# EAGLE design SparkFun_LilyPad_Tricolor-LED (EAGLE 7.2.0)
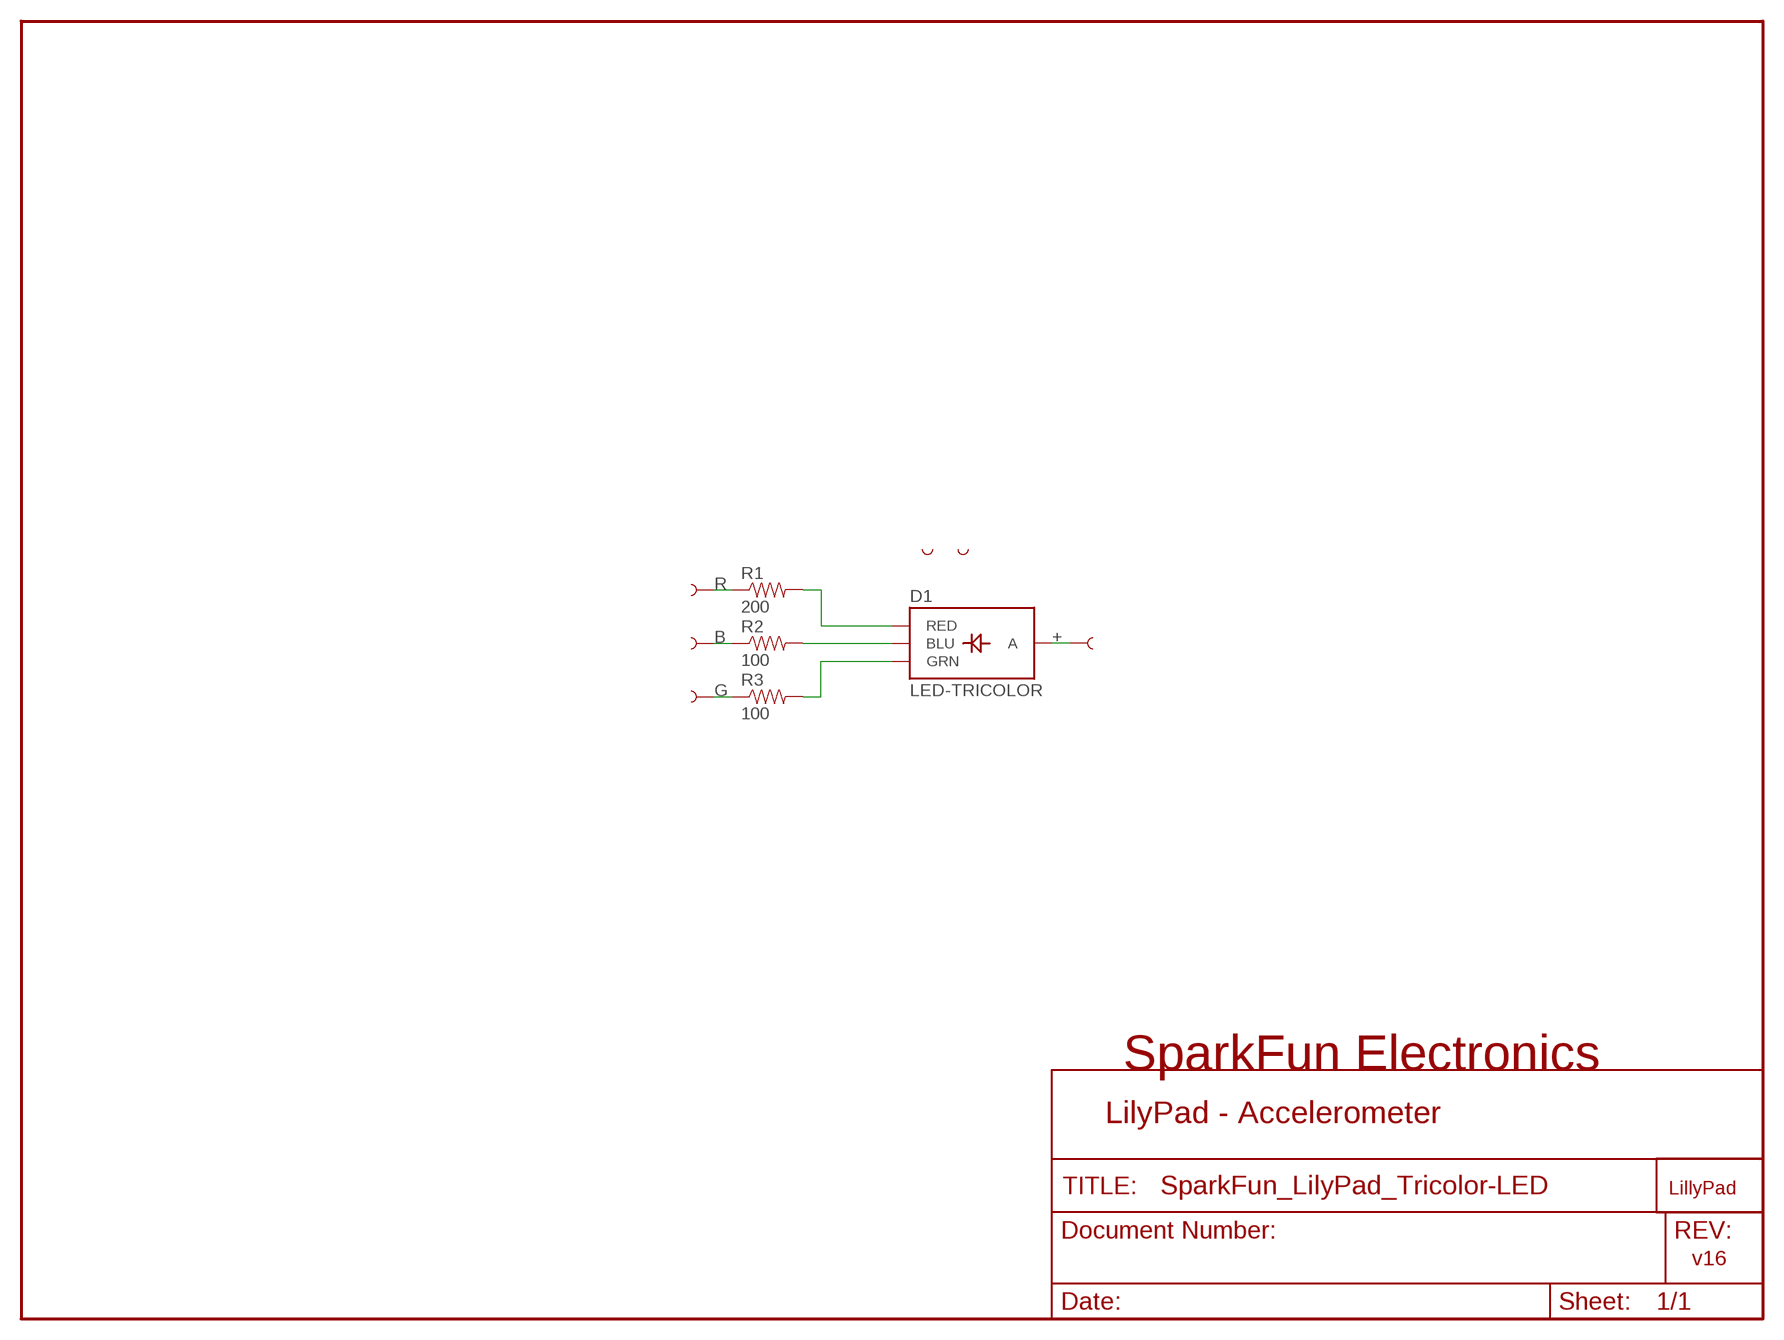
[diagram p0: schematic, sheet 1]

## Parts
D1  LED-TRICOLOR  [LED-TRICOLOR-SMD]
R1  200  RESISTOR0402-RES  [0402-RES]
R2  100  RESISTOR0402-RES  [0402-RES]
R3  100  RESISTOR0402-RES  [0402-RES]
U$1  LOGO-LPL  [LOGO-L]
U$2  SEWTAP-NOHOLE2  [PETAL-NOHOLE-2SIDE]
U$3  SEWTAP-NOHOLE2  [PETAL-NOHOLE-2SIDE]
U$7  SEWTAP6  [PETAL-SMALL-2SIDE]
U$8  SEWTAP6  [PETAL-SMALL-2SIDE]
U$9  SEWTAP6  [PETAL-SMALL-2SIDE]
U$10  SEWTAP6  [PETAL-SMALL-2SIDE]

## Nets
+: D1.A U$10.1
B: R2.1 U$9.1
BLU: D1.B(BLU) R2.2
G: R3.1 U$8.1
GRN: D1.G(GRN) R3.2
R: R1.1 U$7.1
RED: D1.R(RED) R1.2

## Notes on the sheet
- SparkFun Electronics
- LilyPad - Accelerometer
- v16

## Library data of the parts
D1 = SparkFun:LED-TRICOLOR: Tri-Color LED SMD Proven layout and schematic for triple color LED in SMD package - common anode. Spark Fun Electronics SKU : COM-07844
R1-R3 = SparkFun:RESISTOR: Resistor
U$1 = LilyPad-Wearables:LOGO-LP
U$2 U$3 = LilyPad-Wearables:SEWTAP-NOHOLE
U$7-U$10 = LilyPad-Wearables:SEWTAP

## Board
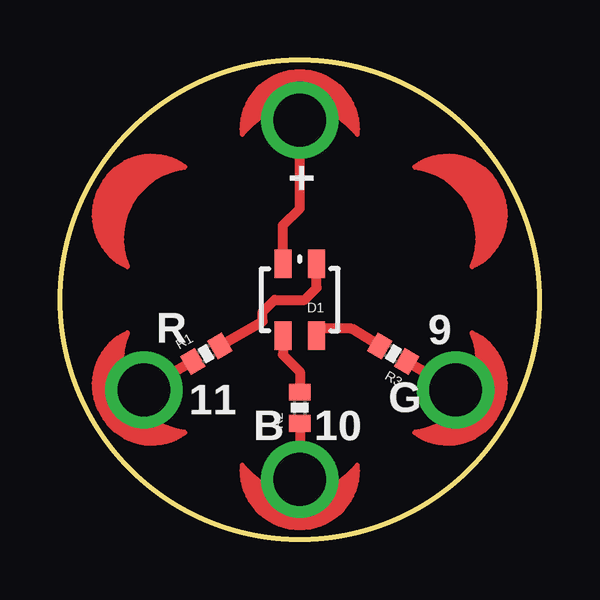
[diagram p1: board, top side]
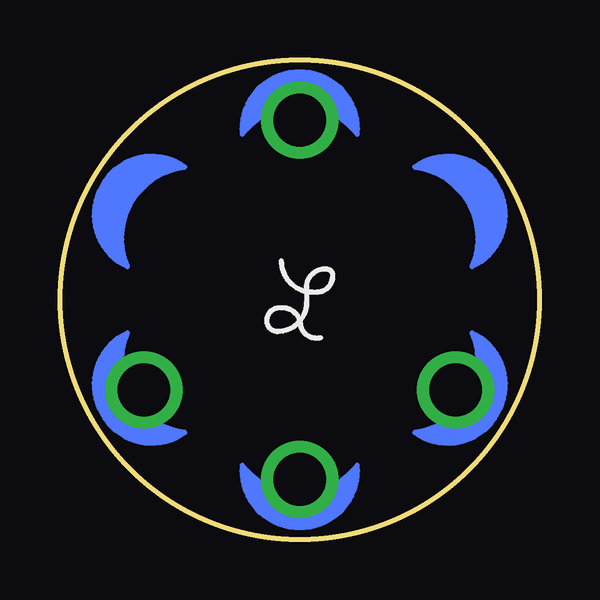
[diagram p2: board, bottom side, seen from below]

Size 20 x 20 mm. Coordinates in mm from the lower left corner, seen from the top.
Outline: circle at 10,10 radius 10
Copper layers (1*16): Top 0.035mm / dielectric 1.5mm / Bottom 0.035mm
Design rules "SparkFun": minimum track width 8mil, minimum drill 20mil, track to track 8mil, track to pad 8mil, pad to pad 8mil, via to via 8mil, smd to smd 8mil, copper to edge 8mil, drill to drill 8mil, minimum pad ring 12mil, minimum via ring 10mil, stop-mask expansion 4mil, vias tented up to drill 20mil, thermal gap 10mil

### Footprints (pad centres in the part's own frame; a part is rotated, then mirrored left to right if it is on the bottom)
LED-TRICOLOR-SMD = smd 0.7 x 1.2: A 0.7,-1.5; B 0.7,1.5; G -0.7,1.5; R -0.7,-1.5
0402-RES = smd 0.7 x 0.9: 1 -0.65,0; 2 0.65,0
PETAL-SMALL-2SIDE = drill 2.2: 1 0,0

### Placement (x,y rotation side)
D1  10,10 180 top
R1  6.1,7.75 30 top
R2  10,5.5 90 top
R3  13.9,7.75 150 top
U$1  10,10 0 bottom
U$2  16.5,13.76 120 top
U$3  3.5,13.76 240 top
U$7  3.5,6.24 300 top
U$8  16.5,6.24 60 top
U$9  10,2.51 0 top
U$10  10,17.49 180 top

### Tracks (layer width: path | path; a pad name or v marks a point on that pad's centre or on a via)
+
  Top 0.406: D1.A 9.3,13.11 10,13.81 U$10.1 10,17.62
B
  Top 0.406: 10,2.45 U$9.1 R2.1
BLU
  Top 0.406: D1.B 9.3,7.7 10,7 R2.2 10.05,6.1
G
  Top 0.406: U$8.1 R3.1
GRN
  Top 0.406: R3.2 12.15,8.8 10.65,8.8 10.65,8.5 D1.G
R
  Top 0.406: U$7.1 3.45,6.25 R1.1
RED
  Top 0.406: R1.2 8.45,9.1 8.45,9.5 8.95,10 10.2,10 10.7,10.5 D1.R

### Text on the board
tPlace: + | R | 9 | 11 | G | B | 10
